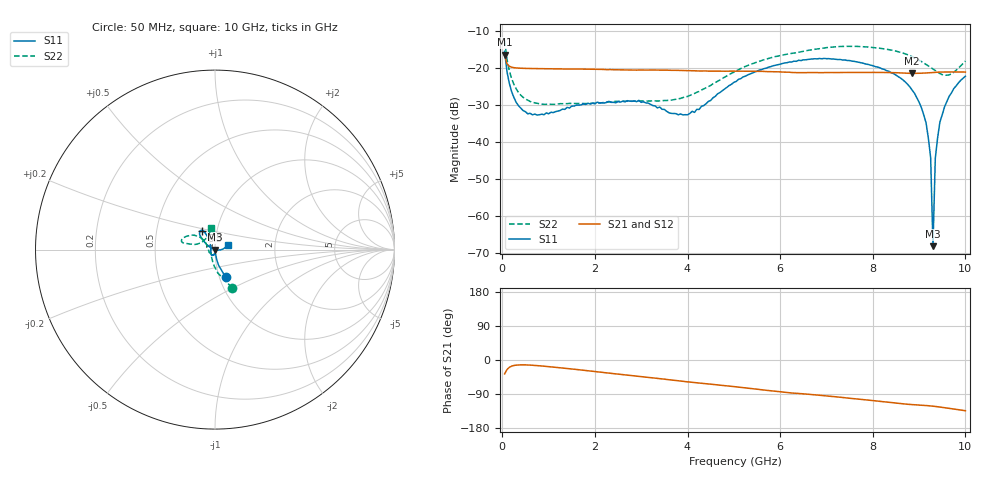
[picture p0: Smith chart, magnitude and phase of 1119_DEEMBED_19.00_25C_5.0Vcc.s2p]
!Hittite Microwave Corp.
!Digital Attenuator/PhaseShifter Rev 1.4.0
!Filename: C:\DATA\DATA\1119_DEEMBED_19.00_25C_5.0Vcc.s2p
!VNA ID: Agilent Technologies,N5224A,MY51441122,A.10.45.03
!Device type:
!2 Port Calibration.
!Temp(C): 25
!Lot Number:
!Serial Number:
!Operator:
!Misc:
!Attenuator:  19.000
# GHZ S DB R 50.0
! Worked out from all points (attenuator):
!   200 points, 50 MHz to 10 GHz, reference 50 ohm
!   highest |S21| = -16.46 dB at 50 MHz (marker M1); lowest = -21.5 dB at 8.85 GHz (marker M2)
!   lowest |S11| = -68.0 dB at 9.3 GHz (marker M3), VSWR 1.00, Z = 50 - j0.0217 ohm
!   |S11| at or under -10 dB: start of sweep to end of sweep
!   |S22| runs from -29.9 to -12.7 dB; largest |S21 - S12| = 0.00026
!   S11 on the Smith chart (normalised r, x): 50 MHz: 1.07, -0.34; 6.5 GHz: 0.85, +0.18; 10 GHz: 1.15, +0.07
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0.05  -15.57 -68.9  -16.46 -36.7  -16.47 -36.7  -12.67 -65.9
0.1  -20.97 -77.0  -18.91 -25.5  -18.91 -25.6  -17.61 -83.0
0.2  -26.39 -80.7  -19.86 -16.3  -19.86 -16.3  -22.88 -99.8
0.55  -32.42 -84.3  -20.21 -13.2  -20.21 -13.1  -28.77 -125.2
1.75  -29.75 -111.3  -20.38 -27.1  -20.39 -27.1  -29.64 -138.8
2.95  -28.80 -123.8  -20.62 -42.8  -20.63 -42.9  -28.98 -157.8
3.4  -30.59 -142.4  -20.65 -49.1  -20.65 -49.1  -28.92 -171.1
4  -32.69 168.7  -20.81 -57.5  -20.82 -57.6  -27.75 164.7
5.05  -23.71 121.2  -20.94 -70.8  -20.95 -70.8  -20.84 140.1
6.5  -17.89 123.8  -21.33 -89.2  -21.34 -89.2  -15.57 152.4
6.7  -17.68 125.7  -21.31 -91.5  -21.32 -91.5  -15.12 154.8
8.35  -20.98 141.3  -21.31 -111.9  -21.31 -111.9  -15.14 167.9
8.85  -26.04 148.3  -21.53 -117.6  -21.53 -117.6  -17.03 167.4
9.05  -30.75 154.8  -21.48 -119.2  -21.49 -119.2  -18.34 166.4
9.15  -34.81 159.5  -21.42 -120.1  -21.44 -120.1  -19.11 164.8
9.2  -38.95 161.1  -21.38 -120.7  -21.39 -120.7  -19.53 163.5
9.25  -44.22 162.4  -21.35 -121.2  -21.36 -121.3  -19.94 161.7
9.3  -68.04 -33.1  -21.30 -121.9  -21.32 -121.9  -20.34 159.4
9.35  -44.42 -13.6  -21.27 -122.6  -21.29 -122.6  -20.78 156.6
9.45  -34.61 -9.2  -21.18 -124.2  -21.20 -124.1  -21.58 149.1
9.65  -27.69 2.8  -21.15 -127.6  -21.17 -127.6  -21.92 127.1
10  -22.30 21.6  -21.18 -133.9  -21.18 -133.9  -18.21 99.7
